PROGRAM MAIN
VAR
	
motorStatus  : BOOL := TRUE;
doorAtHome  : BOOL := TRUE;
motorOutPut  : BOOL := FALSE;


machine : ARRAY [0..2] OF MachineSetting := [
(machineName:= 'Motor_one', targetSpeed := 1),
(machineName:= 'Motor_two', targetSpeed := 2),
(machineName:= 'Motor_three', targetSpeed := 3)
];

initDone : BOOL := FALSE;
index : INT := 0;

END_VAR


IF  NOT initDone THEN	
	initDone := TRUE;
	FOR index := 0 TO 2 DO
    	machine[index].currentSpeed := (index+1)*20;		
	END_FOR;
END_IF

END_PROGRAM
